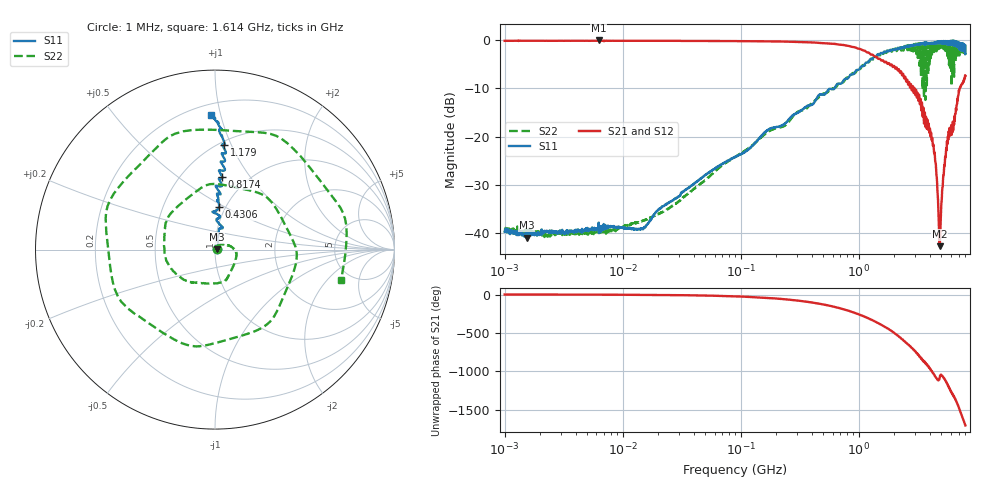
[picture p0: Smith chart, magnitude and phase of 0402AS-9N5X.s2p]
!s-Parameter Generated by FASTRON Sdn. Bhd.
!FASTRON P/N : 0402AS-9N5X
!Keysight Technologies: E5071C_MY46733604_B.14.02
!Date: Mon Dec 01 10:29:48 2025
!Version  :Rev00  Mon Dec 01 10:29:48 2025
!Data & Calibration Information:
!Freq  S11:SOLT2(ON)  S21:SOLT2(ON)  S12:SOLT2(ON)  S22:SOLT2(ON)
!PortZ  Port1:50+j0  Port2:50+j0
!When reading reference impedance value at option line is always used.
! Remarks : This data is being provided solely for informational purposes.
# Hz S dB R 50
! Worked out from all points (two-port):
!   1601 points, 1 MHz to 8 GHz, reference 50 ohm
!   highest |S21| = -0.03 dB at 6.268 MHz (marker M1); lowest = -42.8 dB at 4.856 GHz (marker M2)
!   |S21| within 3 dB of the highest: start of sweep to 1.319 GHz
!   lowest |S11| = -41.0 dB at 1.541 MHz (marker M3), VSWR 1.02, Z = 50.9 + j0.0983 ohm
!   |S11| at or under -10 dB: start of sweep to 621 MHz
!   |S22| runs from -41.0 to -0.5 dB; largest |S21 - S12| = 0.017
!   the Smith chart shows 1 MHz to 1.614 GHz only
!   S11 on the Smith chart (normalised r, x): 1 MHz: 1.02, +0.00; 430.6 MHz: 0.93, +0.47; 817.4 MHz: 0.77, +0.75; 1.179 GHz: 0.53, +0.94; 1.614 GHz: 0.27, +0.93
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1000000  -39.80 7.8  -0.11 -0.2  -0.09 -0.3  -39.40 8.1
1541011  -41.00 6.2  -0.10 -0.5  -0.08 -0.5  -39.80 -0.7
4479405  -39.40 15.5  -0.10 -1.2  -0.09 -1.2  -40.20 17.1
6268472  -37.90 14.8  -0.03 -1.6  -0.04 -1.7  -39.70 15.3
2.00676e7  -35.20 40.0  -0.11 -5.4  -0.10 -5.3  -36.10 46.7
8.994653e7  -24.20 80.3  -0.16 -23.6  -0.15 -23.6  -24.20 25.5
4.006501e8  -13.40 90.4  -0.43 -104.0  -0.42 -104.0  -13.10 -125.0
4.305659e8  -12.50 84.7  -0.48 -112.0  -0.47 -112.0  -12.40 -135.0
8.173602e8  -7.78 84.4  -1.16 149.0  -1.14 149.0  -7.75 31.6
1.179402e9  -4.63 85.1  -2.52 56.6  -2.51 56.5  -4.43 -154.0
1.411421e9  -3.27 87.9  -3.43 -0.6  -3.42 -0.7  -3.52 87.0
1.613809e9  -2.51 91.9  -4.23 -48.7  -4.24 -48.8  -2.82 -13.4
1.7949e9  -2.28 94.5  -4.73 -91.2  -4.73 -91.3  -2.46 -99.7
2.114474e9  -1.70 101.0  -5.96 -171.0  -5.95 -171.0  -2.01 94.8
2.486897e9  -1.36 105.0  -7.80 97.8  -7.78 97.7  -2.11 -93.0
2.839031e9  -1.16 111.0  -10.00 22.0  -9.98 21.8  -0.87 110.0
3.203473e9  -0.76 119.0  -12.60 -65.9  -12.60 -66.2  -1.51 -85.8
3.60885e9  -0.88 129.0  -15.30 -153.0  -15.30 -153.0  -1.36 82.2
3.973689e9  -0.55 134.0  -19.00 128.0  -19.00 128.0  -5.19 -71.4
4.856488e9  -0.20 151.0  -42.80 7.6  -42.90 6.8  -1.52 -167.0
5.276366e9  -0.44 175.0  -26.60 -9.3  -26.60 -9.6  -0.50 4.9
8e9  -1.13 -106.0  -7.35 94.7  -7.38 94.4  -3.05 131.0
